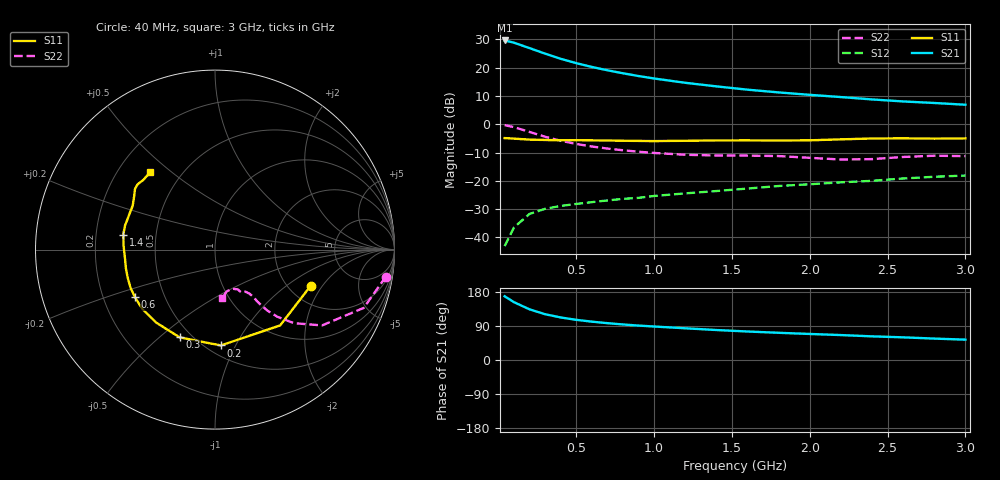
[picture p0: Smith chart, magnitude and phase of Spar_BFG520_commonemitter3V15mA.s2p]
! Filename:  BFG520D.S2P  Version:  2.1
! NXP part #: BFG520  Date: Feb 1992
! Bias condition: Vce=3V, Ic=15mA
! IN LINE PINNING: same data as with cross emitter pinning.
#  MHz  S  MA  R  50
! Freq  S11  S21  S12  S22  !GUM [dB]
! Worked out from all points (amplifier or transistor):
!   21 points, 40 MHz to 3 GHz, reference 50 ohm
!   highest |S21| = 29.6 dB at 40 MHz (marker M1)
!   |S21| within 3 dB of that: start of sweep to 215.3 MHz
!   unconditionally stable (mu >= 1): 1.029 GHz to end of sweep
!   at 300 MHz: K = 0.42, MSG = 27.4 dB, |S12| = -29.9 dB
!   at 1 GHz: K = 0.99, MSG = 20.8 dB, |S12| = -25.4 dB
!   at 3 GHz: K = 1.24, MAG = 9.6 dB, |S12| = -18.1 dB
!   lowest NFmin = 1.30 dB at 500 MHz
!   S11 on the Smith chart (normalised r, x): 40 MHz: 2.61, -1.56; 200 MHz: 0.58, -0.87; 300 MHz: 0.43, -0.59; 600 MHz: 0.34, -0.25; 1.4 GHz: 0.32, +0.07; 3 GHz: 0.34, +0.42
40  0.57 -20.7  30.26 168.2  0.007 80.6  0.964 -9.0
100  0.557 -49.3  27.64 152.7  0.015 71.7  0.89 -21.4
200  0.535 -86.5  22.17 133.7  0.026 58.7  0.731 -35.3
300  0.527 -111.9  17.7 120.8  0.032 52.8  0.601 -43.0
400  0.522 -128.6  14.35 112.3  0.036 50.8  0.511 -47.1
500  0.523 -140.5  12.02 106.0  0.039 49.8  0.449 -49.3
600  0.519 -149.3  10.3 101.2  0.042 50.4  0.404 -50.3
700  0.516 -156.1  8.995 97.2  0.045 51.4  0.372 -50.8
800  0.511 -162.5  7.959 93.8  0.048 52.8  0.347 -51.0
900  0.507 -168.4  7.116 90.8  0.05 54.8  0.327 -51.4
1000  0.504 -173.5  6.441 88.4  0.054 56.2  0.311 -52.0
1200  0.51 177.4  5.404 83.7  0.06 57.9  0.289 -54.2
1400  0.518 170.7  4.671 79.1  0.066 59.6  0.28 -57.0
1600  0.519 165.2  4.085 75.2  0.073 62.1  0.279 -58.4
1800  0.516 158.6  3.653 71.8  0.081 62.6  0.274 -58.9
2000  0.52 151.8  3.308 68.7  0.087 64.3  0.255 -60.3
2200  0.541 146.3  3.024 65.8  0.094 64.3  0.238 -66.3
2400  0.56 142.7  2.747 62.4  0.1 65.9  0.242 -74.5
2600  0.564 139.8  2.528 59.8  0.11 66.1  0.264 -79.5
2800  0.557 135.8  2.377 56.5  0.118 65.0  0.278 -80.4
3000  0.562 130.1  2.212 53.7  0.124 66.2  0.273 -81.2
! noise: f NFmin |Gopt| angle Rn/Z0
500  1.3  0.161  31  0.21
900  1.45  0.155  63  0.2
1000  1.5  0.16  67  0.23
2000  2.05  0.23  165  0.14
